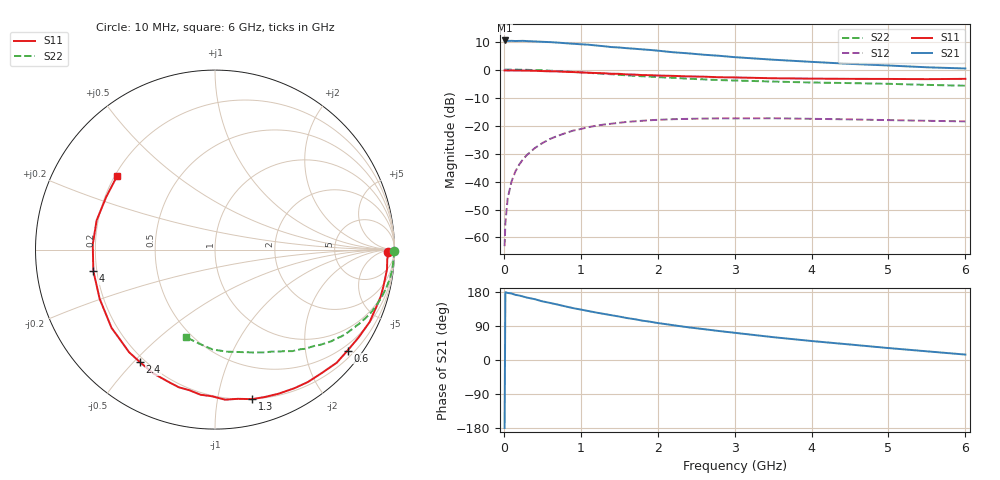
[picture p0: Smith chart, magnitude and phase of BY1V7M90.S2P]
! SIEMENS Small Signal Semiconductors
! BFY420
! Si NPN RF SIEGET Grounded Emitter Transistor in MICRO-X
! VCE = 1.75 V  IC = 0.9 mA
! Common Emitter S-Parameters:  October  1996
# GHz  S  MA  R  50
!  f  S11  S21  S12  S22
! GHz  MAG  ANG  MAG  ANG  MAG  ANG  MAG  ANG
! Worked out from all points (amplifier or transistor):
!   36 points, 10 MHz to 6 GHz, reference 50 ohm
!   highest |S21| = 10.4 dB at 10 MHz (marker M1)
!   |S21| within 3 dB of that: start of sweep to 1.718 GHz
!   unconditionally stable (mu >= 1): 4.628 GHz to end of sweep
!   at 250 MHz: K = 0.03, MSG = 21.1 dB, |S12| = -32.0 dB
!   at 1.4 GHz: K = 0.20, MSG = 13.7 dB, |S12| = -19.3 dB
!   at 6 GHz: K = 1.34, MAG = 6.0 dB, |S12| = -18.5 dB
!   S11 on the Smith chart (normalised r, x): 10 MHz: 48, -15; 600 MHz: 0.36, -2.92; 1.3 GHz: 0.20, -1.26; 2.4 GHz: 0.18, -0.52; 4 GHz: 0.19, -0.08; 6 GHz: 0.21, +0.32
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0.01  0.9627 -0.7  3.307 -179.3  0.0007 106.9  0.9999 -0.3
0.02  0.9647 -1.6  3.302 178.8  0.0018 89.7  0.9961 -0.6
0.05  0.9612 -3.3  3.245 177.0  0.005 88.5  0.9976 -1.6
0.1  0.9646 -6.5  3.256 175.5  0.01 85.2  0.9951 -3.2
0.15  0.9613 -9.6  3.231 171.9  0.0151 85.0  0.9947 -4.8
0.25  0.9594 -15.8  3.257 167.5  0.025 80.3  0.9901 -7.9
0.3  0.955 -18.8  3.222 164.7  0.0298 78.5  0.9878 -9.4
0.4  0.9514 -25.0  3.179 160.6  0.0393 74.7  0.978 -12.6
0.5  0.938 -31.4  3.129 154.8  0.0485 70.9  0.9674 -15.5
0.6  0.9283 -37.3  3.088 150.7  0.0576 66.9  0.9539 -18.5
0.9  0.9011 -55.0  2.887 136.9  0.0811 56.0  0.9068 -26.7
1.1  0.8775 -66.2  2.779 129.2  0.0935 49.7  0.8729 -31.8
1.3  0.8584 -76.1  2.611 121.7  0.1041 43.6  0.8382 -36.3
1.8  0.7962 -100.4  2.291 103.9  0.1215 31.0  0.7587 -45.8
2.2  0.7707 -116.3  2.037 91.9  0.1297 22.5  0.7119 -52.6
2.4  0.7539 -123.6  1.945 86.2  0.1316 19.2  0.685 -55.7
2.8  0.7282 -136.9  1.76 76.4  0.1342 12.9  0.6489 -61.2
3.5  0.6987 -156.9  1.499 60.3  0.1348 4.7  0.6097 -70.0
4  0.6882 -170.1  1.371 50.1  0.1318 0.4  0.5869 -76.5
4.5  0.6817 177.5  1.262 40.9  0.1287 -3.2  0.5723 -83.5
5.5  0.6734 154.1  1.097 22.9  0.1215 -6.5  0.532 -99.3
6  0.6821 143.2  1.044 14.3  0.1185 -6.4  0.514 -108.4
